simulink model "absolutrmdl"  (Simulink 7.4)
settings: Solver=ode45  StartTime=0.0  StopTime=500  RelTol=1e-3
libraries: cstblocks x2

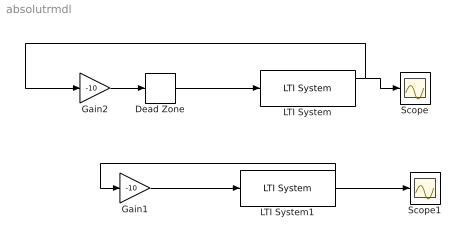
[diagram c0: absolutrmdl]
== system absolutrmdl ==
  Dead Zone : DeadZone  LowerValue=-1  UpperValue=1
  Gain1 : Gain  Gain=-10  ParameterDataType=fixdt(1, 16)  ParameterScaling=2^0  OutDataType=fixdt(1, 16)  OutScaling=2^0
  Gain2 : Gain  Gain=-10  ParameterDataType=fixdt(1, 16)  ParameterScaling=2^0  OutDataType=fixdt(1, 16)  OutScaling=2^0
  LTI System : cstblocks/LTI System  SystemSampleTime=-1  sys=syss  IC=[0 0 0 0.45]
  LTI System1 : cstblocks/LTI System  SystemSampleTime=-1  sys=syss  IC=[0 0 0 0.45]
  Scope : Scope
  Scope1 : Scope
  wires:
  Dead Zone/1 -> LTI System/1
  LTI System/1 -> Scope/1, Gain2/1
  Gain1/1 -> LTI System1/1
  LTI System1/1 -> Gain1/1, Scope1/1
  Gain2/1 -> Dead Zone/1
